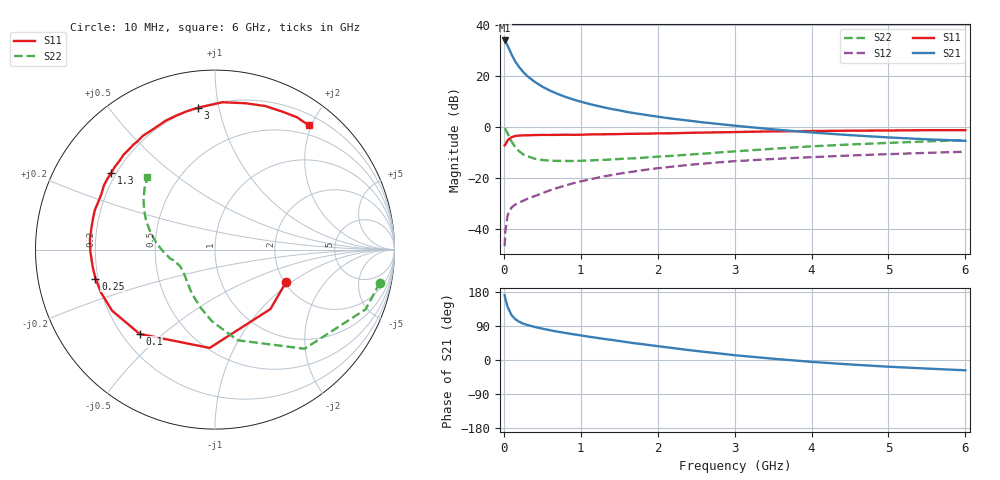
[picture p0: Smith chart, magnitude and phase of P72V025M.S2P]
! SIEMENS Small Signal Semiconductors
! BFP196
! Si NPN RF Bipolar Junction Transistor in SOT143
! VCE = 2 V  IC = 25 mA
! Common Emitter S-Parameters:  May  1996
# GHz  S  MA  R  50
!  f  S11  S21  S12  S22
! GHz  MAG  ANG  MAG  ANG  MAG  ANG  MAG  ANG
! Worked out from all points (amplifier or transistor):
!   36 points, 10 MHz to 6 GHz, reference 50 ohm
!   highest |S21| = 34.1 dB at 10 MHz (marker M1)
!   |S21| within 3 dB of that: start of sweep to 63.04 MHz
!   unconditionally stable (mu >= 1): 578.4 MHz to 3.441 GHz; 3.719 GHz to 4.125 GHz
!   at 250 MHz: K = 0.68, MSG = 25.4 dB, |S12| = -29.1 dB
!   at 1.4 GHz: K = 1.11, MAG = 11.0 dB, |S12| = -18.9 dB
!   at 6 GHz: K = 0.98, MSG = 2.1 dB, |S12| = -9.7 dB
!   S11 on the Smith chart (normalised r, x): 10 MHz: 2.03, -0.92; 100 MHz: 0.27, -0.42; 250 MHz: 0.19, -0.12; 1.3 GHz: 0.18, +0.32; 3 GHz: 0.20, +0.86; 6 GHz: 0.35, +1.96
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0.01  0.435 -24.9  50.73 171.0  0.0045 81.8  0.9368 -11.3
0.02  0.4529 -47.0  48.17 161.1  0.009 72.0  0.903 -21.6
0.05  0.5487 -93.1  39.77 139.5  0.0186 57.3  0.7446 -47.9
0.1  0.6301 -131.8  26.91 118.5  0.026 44.3  0.5206 -76.0
0.15  0.6668 -149.3  19.4 107.5  0.0298 42.0  0.3994 -92.5
0.2  0.6785 -159.2  15.09 100.8  0.0326 42.8  0.3326 -104.1
0.25  0.6851 -166.4  12.19 96.1  0.0352 43.7  0.2903 -113.5
0.3  0.6879 -171.3  10.25 92.6  0.0382 46.1  0.2676 -120.2
0.4  0.6948 -179.3  7.791 87.3  0.0436 49.2  0.2381 -130.6
0.5  0.6992 175.2  6.238 82.9  0.0496 51.7  0.2239 -138.0
0.6  0.6989 170.3  5.214 78.6  0.0568 53.7  0.2179 -143.2
0.7  0.7015 165.4  4.483 74.7  0.0635 54.6  0.2152 -147.1
0.9  0.7024 157.6  3.496 68.1  0.078 55.5  0.214 -153.0
1.1  0.7146 150.2  2.876 61.7  0.0919 55.2  0.2194 -156.8
1.3  0.7196 143.4  2.442 55.7  0.1067 53.9  0.2254 -160.4
1.7  0.7357 130.7  1.872 44.2  0.1336 50.1  0.2423 -166.4
2.2  0.7547 116.8  1.453 31.4  0.1666 44.2  0.2715 -173.5
3  0.796 97.0  1.064 12.6  0.2123 33.7  0.3311 173.0
3.5  0.8219 87.1  0.9 3.4  0.2349 27.2  0.3729 164.8
4.5  0.8475 70.7  0.692 -11.8  0.2749 15.6  0.453 150.7
5.5  0.8673 58.3  0.573 -22.6  0.31 4.8  0.5212 138.8
6  0.8674 53.0  0.535 -27.2  0.3264 -1.0  0.5515 133.0
